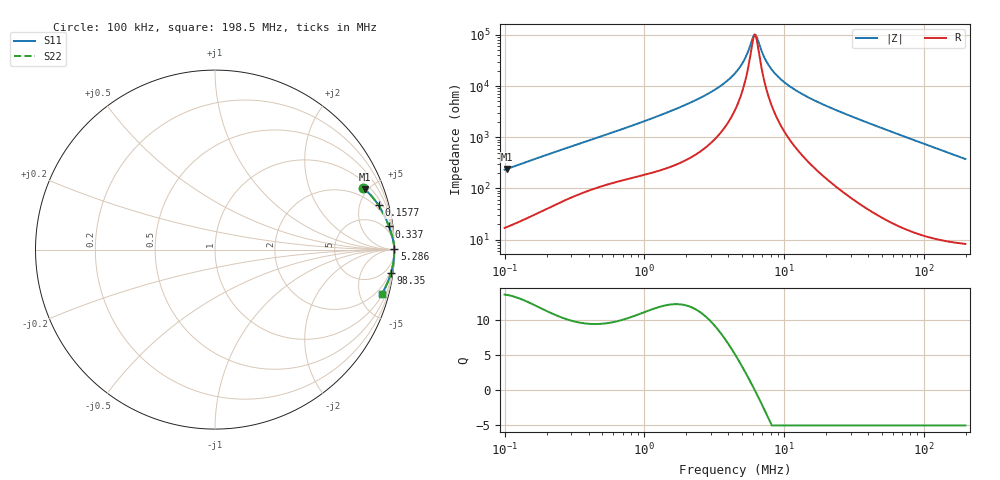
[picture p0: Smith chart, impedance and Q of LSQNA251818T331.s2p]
! LSQNA251818T331  S-PARAMETER MODEL  ( General Type )
! Model Generated by TAIYO YUDEN Corporation (http://www.ty-top.com)
! Version 2.0
! TAIYO YUDEN Control No. 100810NF25SB-FKC
! Copyright(c) 2007 TAIYO YUDEN CO.,LTD. All Rights Reserved.
! Product Description (link to TY-COMPAS)
! https://ds.yuden.co.jp/TYCOMPAS/or/detail?pn=LSQNA251818T331K&u=M
! Products Name : Inductors
! Characteristics :
!  Inductance : 330 uH , SRF(min) : 4.5 MHz , DC Resistance(max) : 9.1 Ohm
!  Rated Current : Saturation :40 mA , Temp Rise : 140 mA (40 degC)
!  Case Size : 2.5 x 1.8 / 0.098 x 0.071 [mm/inch] , Thickness : 1.8 / 0.071 [mm/inch]
!  (Conditions: Temperature = 25 degC , DC Bias Current/Voltage = 0A / 0V)
! External Node Assignments :
!  1  o---GGG---o  2
! GND o---------o GND
! Frequency Range : 0.1MHz  -  198.534594MHz  [ 402 STEP ]
# MHz S RI R 50
! Freq[MHz].  S11 Real  S11 Imag  S21 Real  S21 Imag  S12 Real  S12 Imag  S22 Real  S22 Imag
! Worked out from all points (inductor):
!   401 points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, 100 kHz to 198.5 MHz, reference 50 ohm
!   read as one part in series: L = 365 uH near 103.9 kHz
!   highest Q = 13.6 at 103.9 kHz (marker M1), where L = 367 uH
!   self-resonance near 6.153 MHz
!   S11 on the Smith chart (normalised r, x): 100 kHz: 1.34, +4.61; 157.7 kHz: 1.58, +7.18; 337 kHz: 3, +15; 5.286 MHz: open; 98.35 MHz: 1, -15; 198.5 MHz: 1.16, -7.50
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0.1  0.8251 0.345  0.1749 -0.345  0.1749 -0.345  0.8251 0.345
0.10387  0.8346 0.3365  0.1654 -0.3365  0.1654 -0.3365  0.8346 0.3365
0.157714  0.9113 0.2466  0.0887 -0.2466  0.0887 -0.2466  0.9113 0.2466
0.337019  0.969 0.1291  0.031 -0.1291  0.031 -0.1291  0.969 0.1291
0.356769  0.9713 0.1229  0.0287 -0.1229  0.0287 -0.1229  0.9713 0.1229
1.272844  0.9954 0.0375  0.00459 -0.0375  0.00459 -0.0375  0.9954 0.0375
2.879337  0.9984 0.0139  0.00156 -0.0139  0.00156 -0.0139  0.9984 0.0139
3.755924  0.9988 0.00859  0.00124 -0.00859  0.00124 -0.00859  0.9988 0.00859
4.541117  0.9989 0.00519  0.0011 -0.00519  0.0011 -0.00519  0.9989 0.00519
5.285906  0.999 0.00261  0.00102 -0.00261  0.00102 -0.00261  0.999 0.00261
5.923617  0.999 0.000711  0.000987 -0.000711  0.000987 -0.000711  0.999 0.000711
6.152847  0.999 8.11e-05  0.000978 -8.11e-05  0.000978 -8.11e-05  0.999 8.11e-05
6.270768  0.999 -0.000234  0.000974 0.000234  0.000974 0.000234  0.999 -0.000234
6.513432  0.999 -0.000863  0.000967 0.000863  0.000967 0.000863  0.999 -0.000863
7.027296  0.999 -0.00213  0.000958 0.00213  0.000958 0.00213  0.999 -0.00213
7.439128  0.999 -0.00308  0.000954 0.00308  0.000954 0.00308  0.999 -0.00308
8.65922  0.999 -0.00569  0.000959 0.00569  0.000959 0.00569  0.999 -0.00569
11.08303  0.999 -0.0102  0.00101 0.0102  0.00101 0.0102  0.999 -0.0102
15.89665  0.9988 -0.0181  0.00124 0.0181  0.00124 0.0181  0.9988 -0.0181
56.71438  0.9931 -0.0747  0.00689 0.0747  0.00689 0.0747  0.9931 -0.0747
98.35271  0.981 -0.1289  0.019 0.1289  0.019 0.1289  0.981 -0.1289
198.5346  0.9289 -0.2462  0.0711 0.2462  0.0711 0.2462  0.9289 -0.2462
